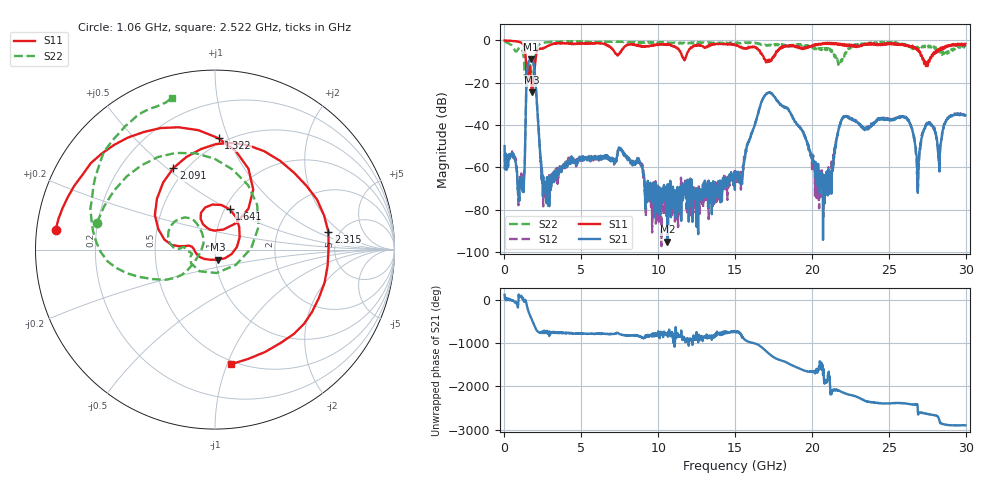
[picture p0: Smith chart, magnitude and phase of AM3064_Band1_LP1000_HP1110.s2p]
# Hz S DB R 50.0
!freq dBS11 angS11 dBS21 angS21 dBS12 angS12 dBS22 angS22
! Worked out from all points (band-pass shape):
!   1600 points, 10 MHz to 29.98 GHz, reference 50 ohm
!   highest |S21| = -8.90 dB at 1.716 GHz (marker M1); lowest = -95.1 dB at 10.6 GHz (marker M2)
!   |S21| within 3 dB of the highest: 1.514 GHz to 1.911 GHz (397.2 MHz wide, 23.2 % of centre)
!   lowest |S11| = -24.6 dB at 1.772 GHz (marker M3), VSWR 1.12, Z = 51.3 - j5.83 ohm
!   |S11| at or under -10 dB: 1.393 GHz to 2.008 GHz (615.6 MHz wide, 36.2 % of centre); 27.28095 GHz to 27.34994 GHz (68.99 MHz wide, 0.253 % of centre); 27.36 GHz to 27.57 GHz (204.7 MHz wide, 0.745 % of centre)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
!   |S22| runs from -22.8 to -0.4 dB; largest |S21 - S12| = 0.0052
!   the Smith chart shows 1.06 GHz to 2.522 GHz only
!   S11 on the Smith chart (normalised r, x): 1.06 GHz: 0.06, +0.06; 1.322 GHz: 0.46, +0.92; 1.641 GHz: 1.06, +0.50; 2.091 GHz: 0.43, +0.53; 2.315 GHz: 4.07, +1.35; 2.522 GHz: 0.47, -1.03
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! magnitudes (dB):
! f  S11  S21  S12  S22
! 10 MHz  0.0  -50.0  -53.3  -0.4
! 1.06 GHz  -1.0  -66.6  -69.2  -3.4
! 1.322 GHz  -4.1  -57.7  -57.9  -16.8
! 1.641 GHz  -12.4  -9.4  -9.3  -11.1
! 1.716 GHz  -18.2  -8.9  -8.9  -13.0
! 1.772 GHz  -24.6  -9.1  -9.0  -16.8
! 2.091 GHz  -5.8  -27.3  -27.3  -3.9
! 2.315 GHz  -3.9  -52.5  -52.7  -1.6
! 2.522 GHz  -3.8  -64.4  -78.5  -1.1
! 5.015 GHz  -1.5  -55.1  -56.3  -0.8
! 7.582 GHz  -5.4  -51.1  -51.8  -0.6
! 10 GHz  -2.0  -79.0  -85.0  -0.9
! 10.6 GHz  -2.0  -95.1  -72.0  -1.0
! 15 GHz  -2.3  -64.9  -67.4  -1.4
! 17.16 GHz  -9.7  -24.8  -24.7  -2.5
! 19.99 GHz  -2.9  -55.9  -55.8  -3.2
! 20.87 GHz  -1.3  -63.6  -64.3  -4.4
! 22.05 GHz  -2.3  -36.0  -35.9  -8.0
! 25 GHz  -1.3  -37.7  -37.4  -1.0
! 26.89 GHz  -4.4  -72.1  -69.7  -3.6
! 27.45 GHz  -11.1  -39.4  -39.4  -2.6
! 29.98 GHz  -1.7  -35.4  -35.6  -3.1
